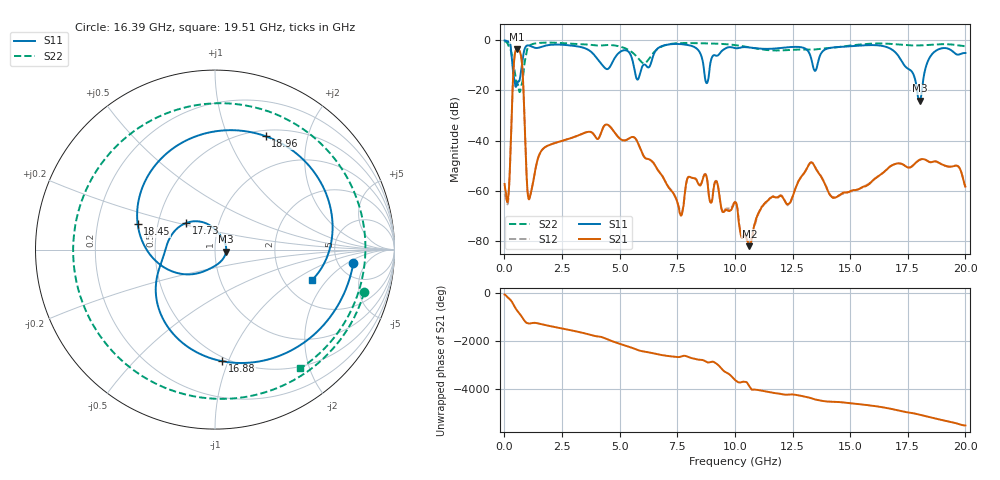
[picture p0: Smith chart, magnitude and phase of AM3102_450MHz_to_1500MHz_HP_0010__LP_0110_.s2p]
!Agilent Technologies,E8364B,MY43040894,A.07.50.67
!Agilent E8364B: A.07.50.67
!Date: Thursday, January 11, 2018 05:25:10
!Correction: S11(Full 2 Port(1,2))
!S21(Full 2 Port(1,2))
!S12(Full 2 Port(1,2))
!S22(Full 2 Port(1,2))
!S2P File: Measurements: S11, S21, S12, S22:
# Hz S  dB  R 50
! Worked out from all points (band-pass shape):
!   1601 points, 10 MHz to 20 GHz, reference 50 ohm
!   highest |S21| = -3.53 dB at 559.7 MHz (marker M1); lowest = -82.1 dB at 10.63 GHz (marker M2)
!   |S21| within 3 dB of the highest: 439.6 MHz to 728.4 MHz (288.8 MHz wide, 49.5 % of centre)
!   lowest |S11| = -24.1 dB at 18.01 GHz (marker M3), VSWR 1.13, Z = 56.5 - j1.25 ohm
!   |S11| at or under -10 dB: 351 MHz to 754 MHz (403.1 MHz wide, 73 % of centre); 5.608 GHz to 6.011 GHz (403.7 MHz wide, 6.95 % of centre); 17.36 GHz to 18.31 GHz (950.1 MHz wide, 5.33 % of centre)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
!   |S22| runs from -20.6 to -0.4 dB; largest |S21 - S12| = 0.0019
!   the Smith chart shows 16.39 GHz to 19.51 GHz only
!   S11 on the Smith chart (normalised r, x): 16.39 GHz: 6.91, -2.54; 16.88 GHz: 0.47, -0.95; 17.73 GHz: 0.70, +0.22; 18.45 GHz: 0.38, +0.14; 18.96 GHz: 0.57, +1.38; 19.51 GHz: 2.86, -1.41
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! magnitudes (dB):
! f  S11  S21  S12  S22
! 10 MHz  -0.1  -57.3  -61.1  -0.4
! 184.9 MHz  -0.6  -61.0  -61.4  -2.4
! 409.8 MHz  -14.5  -9.7  -9.7  -10.5
! 559.7 MHz  -17.3  -3.5  -3.5  -17.5
! 747.1 MHz  -10.4  -7.7  -7.7  -17.7
! 1.084 GHz  -2.1  -63.1  -63.1  -2.2
! 3.346 GHz  -2.7  -37.3  -37.4  -1.6
! 6.682 GHz  -3.0  -52.0  -52.0  -3.2
! 7.656 GHz  -1.5  -69.8  -68.7  -1.1
! 8.781 GHz  -17.1  -54.7  -54.6  -1.2
! 10.01 GHz  -3.1  -64.5  -64.3  -1.9
! 10.63 GHz  -2.9  -82.1  -80.4  -2.8
! 13.34 GHz  -8.4  -48.7  -48.7  -3.8
! 16.39 GHz  -2.2  -53.1  -53.1  -1.3
! 16.68 GHz  -3.0  -50.7  -50.6  -1.4
! 16.88 GHz  -4.1  -49.6  -49.5  -1.5
! 17.73 GHz  -13.2  -49.9  -49.9  -2.0
! 18.01 GHz  -24.1  -47.6  -47.7  -2.0
! 18.45 GHz  -6.9  -48.5  -48.6  -1.8
! 18.96 GHz  -3.2  -49.4  -49.3  -1.5
! 19.51 GHz  -4.9  -50.1  -50.1  -1.8
! 20 GHz  -5.1  -58.3  -58.6  -2.3
